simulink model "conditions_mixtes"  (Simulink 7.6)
settings: Solver=ode15s  StartTime=0.0  StopTime=200  RelTol=1e-3
InitFcn:
  | l=0.1;
  | e=0.01;
  | L=0.5;
  | A=l*L;
  | 
  | Cp=444; % capacité calorifique
  | M=5e-2; % masse du cylindre
  | 
  | Tinf=25+273.15;
  | h=17; % coefficient d'échange
  | 
  | V=l*e*L;
  | rho=M/V; % masse volumique
  | T0=20+273.15; % température initiale
  | 
  | q=10; % flux, W/m2
  | m=h/(rho*Cp*e);
  | phi=q/(rho*Cp*e);
StopFcn:
  | close all
  | load temperatures.mat
  | grid
  | xlabel('temps')
  | plot(x(1,:), x(3,:),x(1,:), x(4,:))
  | grid
  | title('Solution numérique et analytique - Système à conditions mixtes')
  | xlabel('temps')
  | ylabel('\theta(t) = T(t) -Tinf')
libraries: fl_lib x9, nesl_utility x5

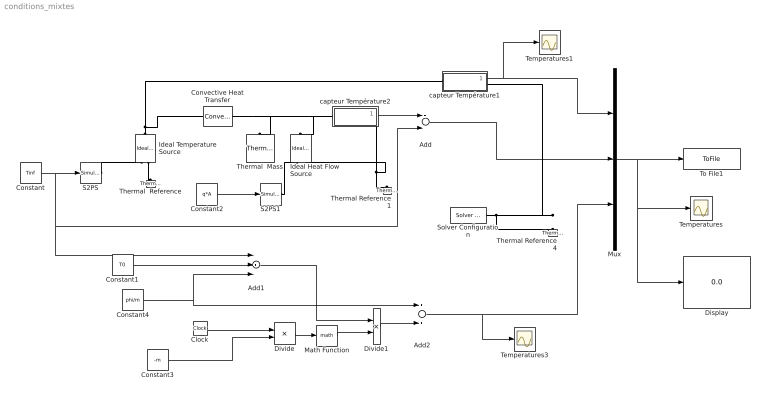
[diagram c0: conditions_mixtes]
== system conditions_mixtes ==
  Add : Sum  Inputs=+-
  Add1 : Sum  Inputs=-+-
  Add2 : Sum  Inputs=2
  Clock : Clock
  Constant : Constant  Value=Tinf
  Constant1 : Constant  Value=T0
  Constant2 : Constant  Value=q*A
  Constant3 : Constant  Value=-m
  Constant4 : Constant  Value=phi/m
  Convective Heat Transfer : fl_lib/Thermal/Thermal Elements/Convective Heat Transfer  DialogController=NetworkEngine.DynNeDlgSource  SystemSampleTime=-1  area=A m^2  heat_tr_coeff=h W/(m^2 * K)  Q_Log=off  T_Log=off  LocalVarNames=|heat_flow|temperature_diff  LocalVarDescs=|Heat flow (J/s)|Temperature difference (K)  LocalVarLogging=[0 0]
  Display : Display
  Divide : Product  Inputs=**
  Divide1 : Product  Inputs=**
  Ideal Heat Flow Source : fl_lib/Thermal/Thermal Sources/Ideal Heat Flow Source  DialogController=NetworkEngine.DynNeDlgSource  SystemSampleTime=-1  Q_Log=off  T_Log=off  LocalVarNames=|Q|T  LocalVarDescs=|Q|T  LocalVarLogging=[0 0]
  Ideal Temperature Source : fl_lib/Thermal/Thermal Sources/Ideal Temperature Source  DialogController=NetworkEngine.DynNeDlgSource  SystemSampleTime=-1  Q_Log=off  T_Log=off  LocalVarNames=|Q|T  LocalVarDescs=|Q|T  LocalVarLogging=[0 0]
  Math Function : Math
  Mux : Mux  Inputs=3
  S2PS : nesl_utility/Simulink-PS Converter  DialogController=NetworkEngine.DynNeUtilDlgSource  SystemSampleTime=-1  PhysicalDomain=network_engine_domain  LeftPortType=input  RightPortType=output  SubClassName=ps_input  Unit=1  AffineConversion=off  InputFilterTimeConstant=.001  UdotUserProvided=0
  S2PS1 : nesl_utility/Simulink-PS Converter  DialogController=NetworkEngine.DynNeUtilDlgSource  SystemSampleTime=-1  PhysicalDomain=network_engine_domain  LeftPortType=input  RightPortType=output  SubClassName=ps_input  Unit=1  AffineConversion=off  InputFilterTimeConstant=.001  UdotUserProvided=0
  Solver Configuration : nesl_utility/Solver Configuration  DialogController=NetworkEngine.DynNeUtilDlgSource  SystemSampleTime=-1  PhysicalDomain=network_engine_domain  LeftPortType=input  RightPortType=generic  SubClassName=solver  Accelerate=off  Profile=off  ResidualTolerance=1e-9  MaxNonlinIter=12  MaxModeIter=2  DoFixedCost=off  UseLocalSampling=off  DoDC=off  LinearAlgebra=Sparse  LocalSolverSampleTime=.001  LocalSolverChoice=NE_BACKWARD_EULER_ADVANCER  UseLocalSolver=off
  Temperatures : Scope
  Temperatures1 : Scope
  Temperatures3 : Scope
  Thermal  Mass : fl_lib/Thermal/Thermal Elements/Thermal Mass  DialogController=NetworkEngine.DynNeDlgSource  SystemSampleTime=-1  mass=M kg  sp_heat=Cp J/kg/K  init_temp=T0 K  Q_Log=off  LocalVarNames=|heat_flow|temperature  LocalVarDescs=|Heat flow (J/s)|Mass temperature (K)  LocalVarLogging=[0 0]
  Thermal  Reference : fl_lib/Thermal/Thermal Elements/Thermal Reference  DialogController=NetworkEngine.DynNeDlgSource  SystemSampleTime=-1  Q_Log=off  LocalVarNames=|Q  LocalVarDescs=|Q  LocalVarLogging=[]
  Thermal Reference1 : fl_lib/Thermal/Thermal Elements/Thermal Reference  DialogController=NetworkEngine.DynNeDlgSource  SystemSampleTime=-1  Q_Log=off  LocalVarNames=|Q  LocalVarDescs=|Q  LocalVarLogging=[]
  Thermal Reference4 : fl_lib/Thermal/Thermal Elements/Thermal Reference  DialogController=NetworkEngine.DynNeDlgSource  SystemSampleTime=-1  Q_Log=off  LocalVarNames=|Q  LocalVarDescs=|Q  LocalVarLogging=[]
  To File1 : ToFile  Filename=temperatures  MatrixName=x
  capteur Température1 : Subsystem
  capteur Température2 : Subsystem
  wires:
  Constant/1 -> S2PS/1, Add/2, Add1/1
  capteur Température1/1(T) -> Mux/1, Temperatures1/1
  Mux/1 -> To File1/1, Temperatures/1, Display/1
  Add/1 -> Mux/2
  capteur Température2/1(T) -> Add/1
  Clock/1 -> Divide/1
  Constant3/1 -> Divide/2
  Divide/1 -> Math Function/1
  Math Function/1 -> Divide1/2
  Constant2/1 -> S2PS1/1
  Constant1/1 -> Add1/2
  Constant4/1 -> Add1/3, Add2/1
  Add1/1 -> Divide1/1
  Divide1/1 -> Add2/2
  Add2/1 -> Mux/3, Temperatures3/1
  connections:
  capteur Température2/LConn1 -- Convective Heat Transfer/RConn1 -- Thermal  Mass/LConn1 -- Ideal Heat Flow Source/LConn1
  Ideal Temperature Source/RConn2 -- Thermal  Reference/LConn1
  Ideal Temperature Source/LConn1 -- capteur Température1/LConn1 -- Convective Heat Transfer/LConn1
  Solver Configuration/RConn1 -- Thermal Reference4/LConn1 -- capteur Température1/RConn1
  S2PS/RConn1 -- Ideal Temperature Source/RConn1
  capteur Température2/RConn1 -- Thermal Reference1/LConn1 -- Ideal Heat Flow Source/RConn2
  S2PS1/RConn1 -- Ideal Heat Flow Source/RConn1

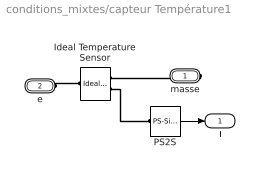
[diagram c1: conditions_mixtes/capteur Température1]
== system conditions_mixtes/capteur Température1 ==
  Ideal Temperature Sensor : fl_lib/Thermal/Thermal Sensors/Ideal Temperature Sensor  DialogController=NetworkEngine.DynNeDlgSource  SystemSampleTime=-1  Qs_Log=off  Ts_Log=off  LocalVarNames=|Qs|Ts  LocalVarDescs=|Qs|Ts  LocalVarLogging=[0 0]
  PS2S : nesl_utility/PS-Simulink Converter  DialogController=NetworkEngine.DynNeUtilDlgSource  SystemSampleTime=-1  PhysicalDomain=network_engine_domain  LeftPortType=input  RightPortType=output  SubClassName=ps_output  Unit=1  AffineConversion=off
  masse : PMIOPort  Port=1  Side=Right
  e : PMIOPort  Port=2  Side=Left
  T : Outport
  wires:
  PS2S/1 -> T/1
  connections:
  Ideal Temperature Sensor/RConn2 -- PS2S/LConn1
  masse/RConn1 -- Ideal Temperature Sensor/RConn1
  e/RConn1 -- Ideal Temperature Sensor/LConn1

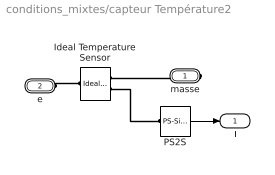
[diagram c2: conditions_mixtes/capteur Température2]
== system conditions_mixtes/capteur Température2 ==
  Ideal Temperature Sensor : fl_lib/Thermal/Thermal Sensors/Ideal Temperature Sensor  DialogController=NetworkEngine.DynNeDlgSource  SystemSampleTime=-1  Qs_Log=off  Ts_Log=off  LocalVarNames=|Qs|Ts  LocalVarDescs=|Qs|Ts  LocalVarLogging=[0 0]
  PS2S : nesl_utility/PS-Simulink Converter  DialogController=NetworkEngine.DynNeUtilDlgSource  SystemSampleTime=-1  PhysicalDomain=network_engine_domain  LeftPortType=input  RightPortType=output  SubClassName=ps_output  Unit=1  AffineConversion=off
  masse : PMIOPort  Port=1  Side=Right
  e : PMIOPort  Port=2  Side=Left
  T : Outport
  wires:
  PS2S/1 -> T/1
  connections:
  e/RConn1 -- Ideal Temperature Sensor/LConn1
  masse/RConn1 -- Ideal Temperature Sensor/RConn1
  Ideal Temperature Sensor/RConn2 -- PS2S/LConn1
